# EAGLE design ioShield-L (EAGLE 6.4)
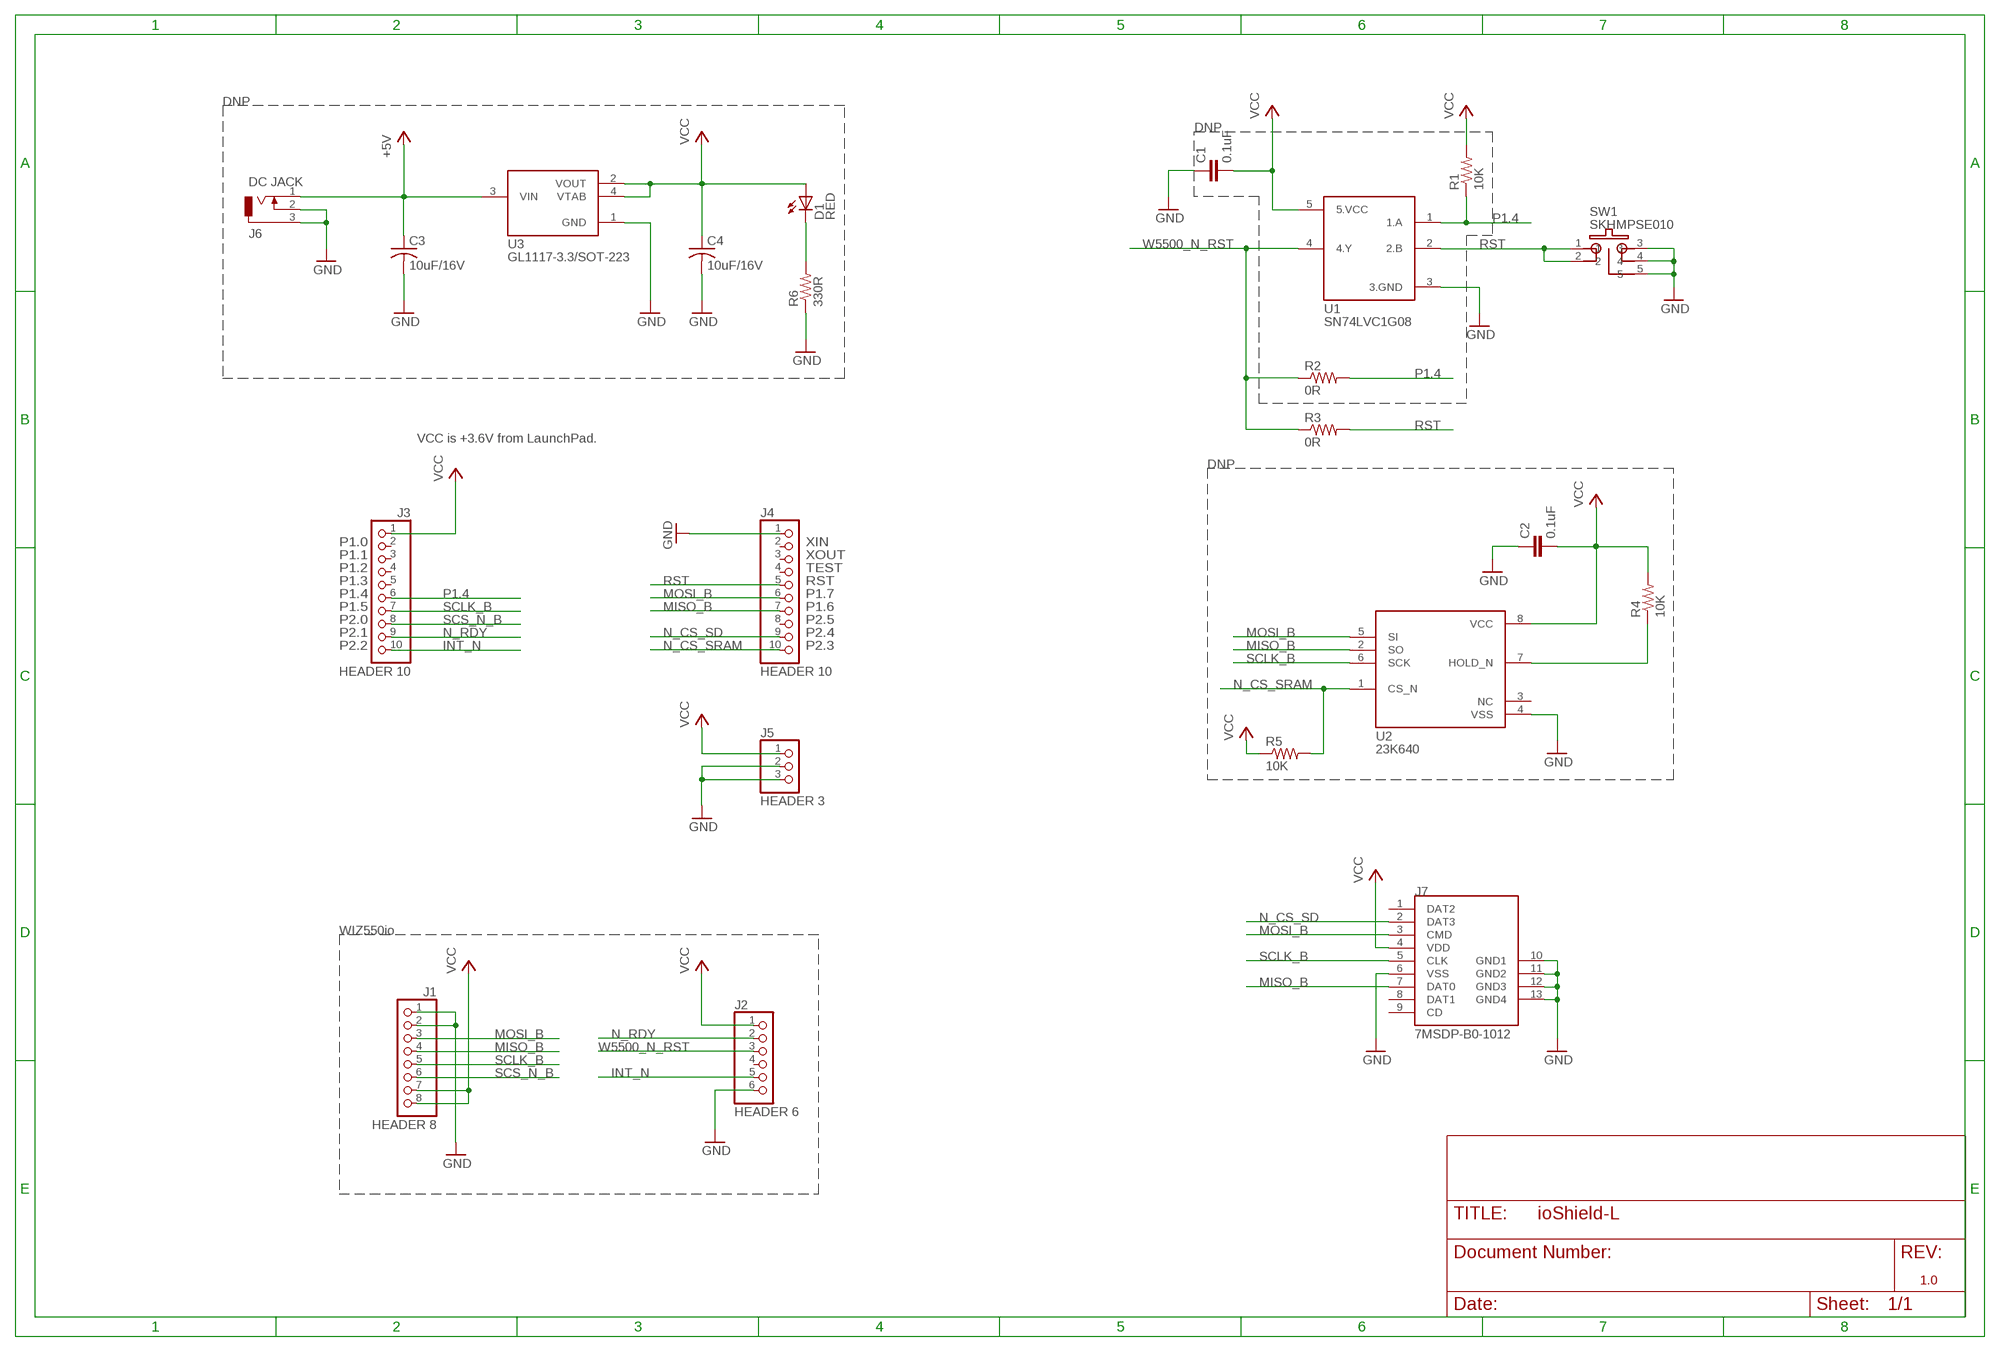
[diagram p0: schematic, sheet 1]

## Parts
C1  0.1uF  C1608  [C1608]
C2  0.1uF  C1608  [C1608]
C3  10uF/16V  CT-A(3216)  [CT-A(3216)]
C4  10uF/16V  CT-A(3216)  [CT-A(3216)]
D1  RED  LED1608  [CHIP-LED1608]
J1  HEADER 8  PINHD-1X8  [1X08]
J2  HEADER 6  PINHD-1X6  [1X06]
J3  HEADER 10  PINHD-1X10  [1X10]
J4  HEADER 10  PINHD-1X10  [1X10]
J5  HEADER 3  PINHD-1X3  [1X03]
J6  DC JACK  DC-005  [DC-005-PACK]
J7  7MSDP-B0-1012  [MICROSD_HC]
R1  10K  R1608  [R1608]
R2  0R  R1608  [R1608]
R3  0R  R1608  [R1608]
R4  10K  R1608  [R1608]
R5  10K  R1608  [R1608]
R6  330R  R1608  [R1608]
SW1  SKHMPSE010  TACT_6.2X6.5  [TACT_6.2X6.5]
U1  SN74LVC1G08  SN74LVC08DBV  [SOT-23-5]
U2  23K640  23K640/SOIC  [SO-08]
U3  GL1117-3.3/SOT-223  [SOT223_HC]

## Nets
+5V: C3.+ J6.1 U3.3(VIN)
GND: C1.1 C2.1 C3.- C4.- J1.1 J1.2 J2.6 J4.1 J5.2 J5.3 J6.2 J6.3 J7.6(VSS) J7.10(GND1) J7.11(GND2) J7.12(GND3) J7.13(GND4) R6.1 SW1.3 SW1.4 SW1.5 U1.3(3.GND) U2.4(VSS) U3.1(GND)
INT_N: J2.5 J3.10
MISO_B: J1.4 J4.7 J7.7(DAT0) U2.2(SO)
MOSI_B: J1.3 J4.6 J7.3(CMD) U2.5(SI)
N$2: R4.1 U2.7(HOLD_N)
N$4: D1.C R6.2
N_CS_SD: J4.9 J7.2(DAT3)
N_CS_SRAM: J4.10 R5.2 U2.1(CS_N)
N_RDY: J2.2 J3.9
P1.4: J3.6 R1.1 R2.2 U1.1(1.A)
RST: J4.5 R3.2 SW1.1 SW1.2 U1.2(2.B)
SCLK_B: J1.5 J3.7 J7.5(CLK) U2.6(SCK)
SCS_N_B: J1.6 J3.8
VCC: C1.2 C2.2 C4.+ D1.A J1.7 J1.8 J2.1 J3.1 J5.1 J7.4(VDD) R1.2 R4.2 R5.1 U1.5(5.VCC) U2.8(VCC) U3.2(VOUT) U3.4(VTAB)
W5500_N_RST: J2.3 R2.1 R3.1 U1.4(4.Y)
Unconnected: J2.4 J3.2 J3.3 J3.4 J3.5 J4.2 J4.3 J4.4 J4.8 J7.1(DAT2) J7.8(DAT1) J7.9(CD) U2.3(NC)

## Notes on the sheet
- DNP
- DNP
- VCC is +3.6V from LaunchPad.
- DNP
- P1.0 | XIN
- P1.1 | XOUT
- P1.2 | TEST
- P1.3 | RST
- P1.4 | P1.7
- P1.5 | P1.6
- P2.0 | P2.5
- P2.1 | P2.4
- P2.2 | P2.3
- WIZ550io
- 1.0

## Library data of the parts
C1 C2 = rlc_HC:C1608: C1608
C3 C4 = rlc_HC:CT-A(3216): CT-A(3216)
D1 = rlc_HC:LED1608: LED 1608
J1 = pinhead:PINHD-1X8: PIN HEADER
J2 = pinhead:PINHD-1X6: PIN HEADER
J3 J4 = pinhead:PINHD-1X10: PIN HEADER
J5 = pinhead:PINHD-1X3: PIN HEADER
J6 = con-jack_HC:DC-005: DC-005
J7 = socket_HC:7MSDP-B0-1012: Micro SD Connector Part No. 7MSDP-B0-1012
R1-R6 = rlc_HC:R1608: R1608
SW1 = switch_HC:TACT_6.2X6.5: ALPS TACT_6.2X6.5
U1 = logic_HC:SN74LVC08DBV: SN74LVC1G08DBV 2Input Single AND Gate
U2 = memory_HC:23K640/SOIC: 23K640 SOIC(SN) Package
U3 = dc-dc:GL1117-3.3/SOT-223: GL1117-3.3/SOT-223

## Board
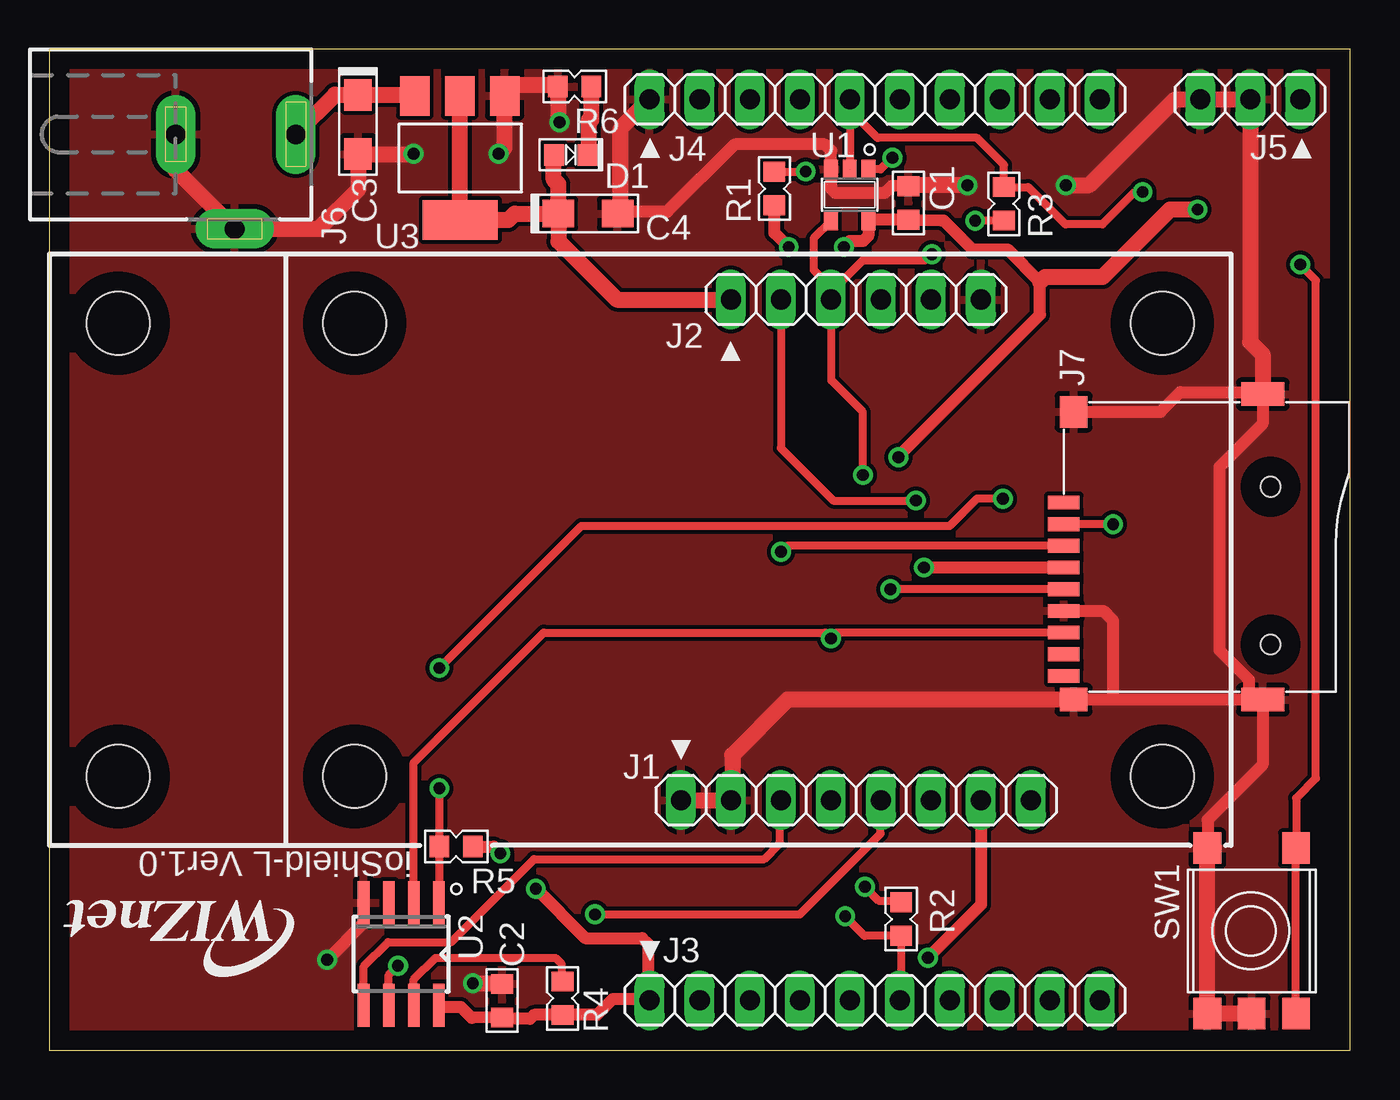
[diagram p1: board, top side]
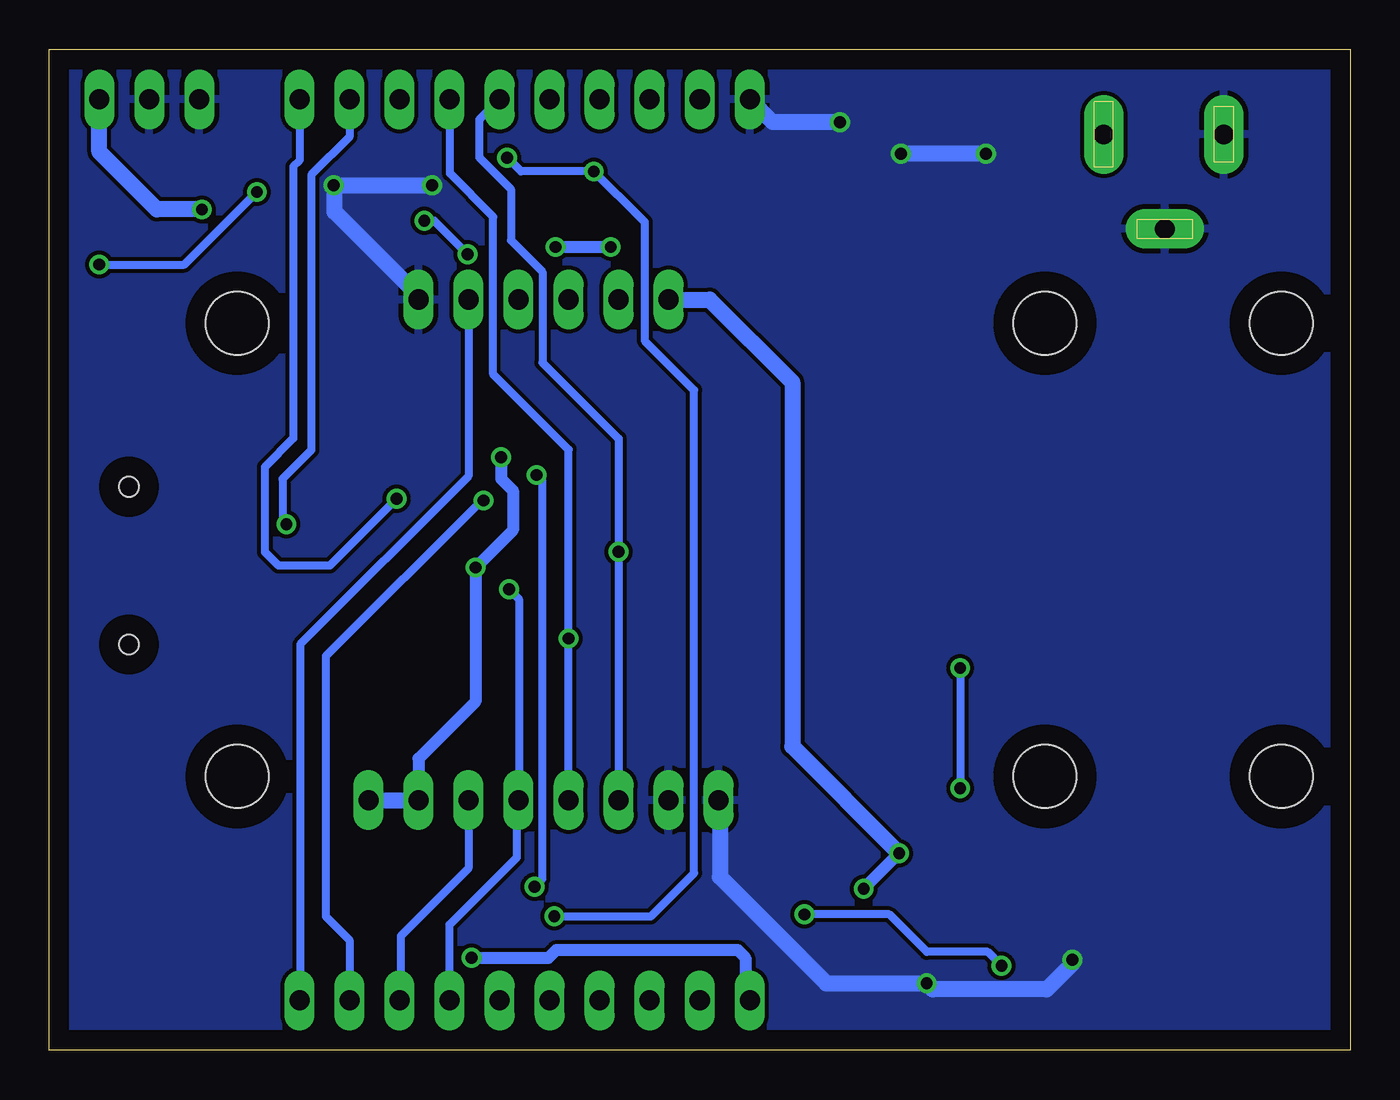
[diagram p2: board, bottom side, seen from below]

Size 66.04 x 50.8 mm. Coordinates in mm from the lower left corner, seen from the top.
Outline: 0,0 66.04,0 66.04,50.8 0,50.8 0,0
Copper layers (1*16): Top 0.035mm / dielectric 1.5mm / Bottom 0.035mm
Design rules "default *": minimum track width 10mil, minimum drill 23mil, track to track 8mil, track to pad 8mil, pad to pad 8mil, via to via 8mil, smd to smd 8mil, copper to edge 40mil, drill to drill 8mil, minimum pad ring 10mil, minimum via ring 8mil, stop-mask expansion 4mil, vias tented up to drill 0mil, thermal gap 10mil
Holes 3.2 mm at 3.5,13.9 56.5,13.9 3.5,36.9 56.5,36.9 15.5,36.9 15.5,13.9

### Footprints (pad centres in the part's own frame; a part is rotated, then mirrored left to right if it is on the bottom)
C1608 = smd 1 x 1.1: 1 -0.85,0; 2 0.85,0
CT-A(3216) = smd 1.6 x 1.4: + -1.5,0; - 1.5,0
CHIP-LED1608 = smd 1 x 1.1: A -0.85,0; C 0.85,0
1X08 = drill 1.016 long: 1 -8.89,0; 2 -6.35,0; 3 -3.81,0; 4 -1.27,0; 5 1.27,0; 6 3.81,0; 7 6.35,0; 8 8.89,0
1X06 = drill 1.016 long: 1 -6.35,0; 2 -3.81,0; 3 -1.27,0; 4 1.27,0; 5 3.81,0; 6 6.35,0
1X10 = drill 1.016 long: 1 -11.43,0; 2 -8.89,0; 3 -6.35,0; 4 -3.81,0; 5 -1.27,0; 6 1.27,0; 7 3.81,0; 8 6.35,0; 9 8.89,0; 10 11.43,0
1X03 = drill 1.016 long: 1 -2.54,0; 2 0,0; 3 2.54,0
DC-005-PACK = drill 1 pad 2 long: 1 0,5.64; 2 0,-0.46; 3 4.8,2.54
MICROSD_HC = smd 0.7 x 1.6: 1 10.6,11.2; 2 9.5,11.2; 3 8.4,11.2; 4 7.3,11.2; 5 6.2,11.2; 6 5.1,11.2; 7 4,11.2; 8 2.9,11.2; 9 1.8,11.2 | smd 1.2 x 1.4: 10 0.6,10.7 | smd 1.6 x 1.4: 11 15.2,10.7 | smd 1.2 x 2.2: 12 16.1,1.1; 13 0.6,1.1 | hole 1: 3.4,0.7; 11.4,0.7
R1608 = smd 1 x 1.1: 1 -0.85,0; 2 0.85,0
TACT_6.2X6.5 = smd 1.6 x 1.4: 1 -4.2,0; 2 4.2,0; 3 -4.2,-4.5; 4 4.2,-4.5; 5 4.2,-2.25
SOT-23-5 = smd 0.69 x 0.99: 1 -0.95,-1.29; 2 0,-1.29; 3 0.95,-1.29; 4 0.95,1.3; 5 -0.95,1.3
SO-08 = smd 0.6 x 2.2: 1 -1.905,-2.6; 2 -0.635,-2.6; 3 0.635,-2.6; 4 1.905,-2.6; 5 1.905,2.6; 6 0.635,2.6; 7 -0.635,2.6; 8 -1.905,2.6
SOT223_HC = smd 1.499 x 2.007: 1 -2.261,-3.15; 2 0.025,-3.15; 3 2.311,-3.15 | smd 3.81 x 2.007: 4 0,3.15

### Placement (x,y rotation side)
C1  43.62,43 270 top
C2  22.99,2.53 270 top
C3  15.68,46.98 270 top
C4  27.35,42.46 0 top
D1  26.47,45.44 0 top
J1  40.95,12.7 0 top
J2  40.95,38.1 0 top
J3  41.91,2.54 0 top
J4  41.91,48.26 0 top
J5  60.96,48.26 180 top
J6  6.87,46.48 270 top
J7  62.7,17.2 90 top
R1  36.81,43.73 270 top
R2  43.24,6.66 270 top
R3  48.46,42.96 90 top
R4  26.06,2.64 270 top
R5  20.66,10.34 180 top
R6  26.67,48.91 0 top
SW1  63.29,6.06 270 top
U1  40.63,43.42 180 top
U2  17.87,4.89 180 top
U3  20.86,45.29 180 top

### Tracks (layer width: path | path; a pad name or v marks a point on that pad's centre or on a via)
+5V
  Top 0.813: J6.1 12.51,46.51 14.5,48.5 15.66,48.5 C3.+ 18.5,48.48 U3.3
GND  (via drill 0.6)
  Top 0.406: 29,42.62 C4.- | 15.6,45.41 C3.- | R6.1
  Top 0.61: C1.1 42.77,43.87 42.4,43.5 39.9,43.5 39.7,43.7 39.7,44.69 U1.3 39.68,45.66 39.37,45.97 34.8,45.97 31.37,42.55 28.93,42.55 C4.- | U2.4 15.96,6.46 v14.1,4.6 | SW1.3 58.8,10.28 58.8,11.7 61.6,14.5 J7.13 60.9,17.8 | 60.9,17.8 54,17.8 | 54,17.8 J7.10 | J7.11 56.4,32.4 57.4,33.4 61.5,33.4 J7.12 61.6,31.8 59.4,29.6 59.4,20.3 60.9,18.8 60.9,17.8 | J7.6 53.5,22.3 54,21.8 54,17.8
  Top 0.813: J6.2 6.41,44.68 J6.3 13.68,41.68 15.7,43.7 15.7,45.46 C3.- 18.48,45.48 v18.5,45.5 | v22.8,45.5 23.1,45.8 23.1,48.42 U3.1 23.12,48.72 23.4,49 25.73,49 R6.1 25.82,47.18 v25.9,47.1 | 29,42.62 29,46.78 J4.1 | v46.6,43.9 43.64,43.9 C1.1 | v21.5,3.4 22.99,3.4 C2.1 | SW1.5 SW1.4 SW1.3 | J7.12 61.59,35.31 60.96,35.94 J5.2 J5.3 57.15,48.26 52.79,43.9 v51.6,43.9 | J1.1 J1.2 34.67,12.77 34.67,14.99 37.48,17.8 J7.10
  Bottom 0.406: 32,12.64 J1.1
  Bottom 0.813: v18.5,45.5 v22.8,45.5 | v25.9,47.1 29.32,47.1 J4.1 | v46.6,43.9 v51.6,43.9 51.56,43.86 51.56,42.55 47.3,38.28 J2.6 | 32,12.64 32,8.8 26.6,3.4 v21.5,3.4 21.2,3.1 15.4,3.1 14.1,4.4 v14.1,4.6
  pour Top: -1,-1 67,-1 67,52 -1,52
  pour Bottom: -1,-1 67,-1 67,52 -1,52
INT_N
  Bottom 0.406: J2.5 44.76,29.14 53.3,20.6 53.3,2.58 J3.10
MISO_B  (via drill 0.6)
  Top 0.406: U2.2 18.5,14.61 25.1,21.2 39.38,21.2 v39.68,20.9 39.98,21.2 J7.7
  Bottom 0.406: J1.4 v39.68,20.9 39.68,30.48 43.5,34.3 43.5,42.3 45.7,44.5 45.7,48.24 J4.7
MOSI_B  (via drill 0.6)
  Top 0.406: U2.5 15.96,4.26 17.2,5.5 20.4,5.5 24.6,9.7 36.3,9.7 37.1,10.5 37.1,12.66 J1.3 | J7.3 37.44,25.6 v37.14,25.3
  Bottom 0.406: 43.2,48.24 J4.6 44.2,47.24 44.2,45.3 42.6,43.7 42.6,41.1 41,39.5 41,34.9 37.14,31.04 v37.14,25.3 J1.3
N$2
  Top 0.406: U2.7 18.5,3.6 19.6,4.7 25.7,4.7 26,4.4 26,3.55 R4.1
N$4
  Top 0.813: D1.C 27.4,45.44 27.4,47.2 27.52,47.2 R6.2
N_CS_SD  (via drill 0.6)
  Top 0.406: v54,26.7 J7.2
  Bottom 0.406: v54,26.7 54.2,26.9 54.2,29 52.74,30.46 52.74,44.42 50.8,46.36 J4.9
N_CS_SRAM  (via drill 0.6)
  Top 0.406: U2.1 19.81,7.52 R5.2 v19.8,13.3 | v48.4,28 47.1,28 45.7,26.6 27,26.6 v19.8,19.4
  Bottom 0.406: v48.4,28 51.8,24.6 54.4,24.6 55.1,25.3 55.1,29.6 53.65,31.05 53.65,44.84 53.34,45.15 J4.10 | v19.8,19.4 v19.8,13.3
N_RDY  (via drill 0.6)
  Top 0.406: J2.2 37.14,30.56 39.8,27.9 v44,27.9
  Bottom 0.406: J3.9 50.8,5.6 52,6.8 52,20 44.1,27.9 v44,27.9
P1.4  (via drill 0.6)
  Top 0.406: J3.6 43.24,2.6 R2.2 41.39,5.81 v40.4,6.8 | 41.6,44.73 U1.1 42.2,44.7 v42.8,45.3 | R1.1 38.38,44.58 v38.4,44.6
  Bottom 0.406: v42.8,45.3 42.1,44.6 v38.4,44.6 37.2,43.4 37.18,43.4 35.81,42.04 35.81,36.01 33.3,33.5 33.3,9 35.5,6.8 v40.4,6.8
RST  (via drill 0.6)
  Top 0.406: J4.5 40.64,47.7 | 40.64,47.7 U1.2 | SW1.2 SW1.1 63.3,10.28 63.3,12.8 64.3,13.8 64.3,39.08 v63.5,39.88 | 40.64,47.7 42.04,46.3 47.1,46.3 48.46,44.94 R3.2 49.69,43.81 51.59,41.91 53.47,41.91 55.12,43.56 v55.5,43.56
  Bottom 0.406: v63.5,39.88 59.18,39.88 v55.5,43.56
SCLK_B  (via drill 0.6)
  Top 0.406: U2.6 17.23,3.83 v17.7,4.3 | v27.7,6.9 38.1,6.9 42.2,11 42.2,12.68 J1.5 | J7.5 v42.7,23.4
  Bottom 0.406: J3.7 45.72,6.38 42.3,9.8 42.3,12.62 J1.5 42.2,12.72 42.2,22.9 v42.7,23.4 | v17.7,4.3 18.4,5 21.5,5 23.4,6.9 v27.7,6.9
SCS_N_B
  Bottom 0.406: J1.6 44.76,9.24 48.2,5.8 48.2,2.6 J3.8
VCC  (via drill 0.6)
  Top 0.406: U1.5 | R4.2 | 30.42,2.6 J3.1 | 36.7,42.77 R1.2
  Top 0.61: J1.7 47.3,7.4 v44.6,4.7 | 30.42,2.6 28.6,2.6 27.8,1.8 R4.2 | R4.2 24.6,1.8 24.4,1.6 23.04,1.6 C2.2 21.45,1.65 20.9,2.2 19.86,2.2 U2.8 | R5.1 22.56,10.34 v22.9,10 | v24.7,8.2 27.2,5.7 30.1,5.7 30.4,5.4 30.4,2.62 J3.1 | J7.4 v44.4,24.5 | v43.1,30.1 43.1,30.15 50.29,37.34 50.29,38.99 48.64,40.64 46.86,40.64 45.4,42.1 45.3,42.1 45.28,42.12 C1.2 41.61,42.15 U1.5 41.58,41.33 41.31,41.06 40.63,41.06 v40.34,40.77 | v37.54,40.77 37.52,40.77 36.81,41.48 R1.2
  Top 0.813: U3.2 20.84,42.16 U3.4 23.31,42.14 23.63,42.46 C4.+ | v58.29,42.67 56.9,42.67 53.47,39.24 50.55,39.24 50.29,38.99 | C4.+ 25.85,43.95 25.61,44.19 D1.A | C4.+ 25.85,41.05 28.81,38.09 34.59,38.09 J2.1
  Bottom 0.61: v44.6,4.7 40.7,4.7 40.3,5.1 31.1,5.1 30.7,4.7 30.7,2.76 J3.1 | v22.9,10 v24.7,8.2 | J1.7 47.3,14.8 44.4,17.7 v44.4,24.5 42.5,26.4 42.5,28.4 43.1,29 v43.1,30.1 | v40.34,40.77 v37.54,40.77
  Bottom 0.813: J1.8 J1.7 | v58.29,42.67 60.58,42.67 63.5,45.59 J5.1 | J2.1 32.51,38.1 28.32,33.91 28.32,15.42 v22.9,10
W5500_N_RST  (via drill 0.6)
  Top 0.406: U1.4 39.68,42.08 38.8,41.2 38.8,39.6 39.2,39.2 39.46,39.2 39.68,38.98 | v41.3,29.2 41.3,32.4 39.7,34 39.7,38.08 J2.3 39.68,38.98 | R3.1 v47.01,42.11 v47,42.1 | 39.68,38.98 40.18,38.98 41.3,40.1 44.5,40.1 v44.8,40.4 | v41.4,8.3 42.1,7.6 43.16,7.6 R2.1
  Bottom 0.406: v47,42.1 46.5,42.1 v44.8,40.4 | v41.4,8.3 41,8.7 41,28.9 v41.3,29.2

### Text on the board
tPlace: ioShield-L Ver1.0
